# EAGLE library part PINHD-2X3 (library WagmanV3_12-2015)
PIN HEADER
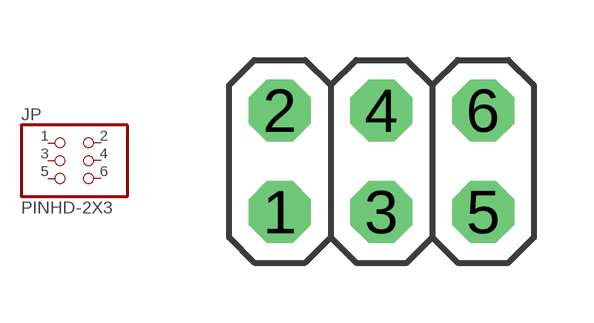
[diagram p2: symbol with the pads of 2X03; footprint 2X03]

Designator prefix JP

## PINHD-2X3  [2X03]
1  1  pas
2  2  pas
3  3  pas
4  4  pas
5  5  pas
6  6  pas

## Footprint 2X03 (pad centres in mm)
PIN HEADER
drill 0.95 pad 1.55 octagon: 1 -2.54,-1.27; 2 -2.54,1.27; 3 0,-1.27; 4 0,1.27; 5 2.54,-1.27; 6 2.54,1.27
